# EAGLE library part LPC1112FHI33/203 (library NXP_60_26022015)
32-bit ARM Cortex-M0 microcontroller; up to 64 kB flash and 8 kB SRAM The LPC1110/11/12/13/14/15 are a ARM Cortex-M0 based, low-cost 32-bit MCU family, designed for 8/16-bit microcontroller applications, offering performance, low power, simple instruction set and memory addressing together with reduced code size compared to existing 8/16-bit architectures. The LPC1110/11/12/13/14/15 operate at CPU frequencies of up to 50 MHz. The peripheral complement of the LPC1110/11/12/13/14/15 includes up to 64 kB of flash memory, up to 8 kB of data memory, one Fast-mode Plus I 2 C-bus interface, one RS-485/EIA-485 UART, up to two SPI interfaces with SSP features, four general purpose counter/timers, a 10-bit ADC, and up to 42 general purpose I/O pins. Remark: The LPC111x series consists of the LPC1100 series (parts LPC111x/101/201/301), LPC1100L series (parts LPC111x/002/102/202/302), and the LPC1100XL series (parts LPC111x/103/203/303/323/333). The LPC1100L and LPC1100XL series include the power profiles, a windowed watchdog timer, and a configurable open-drain mode. AAL Eindhoven MK
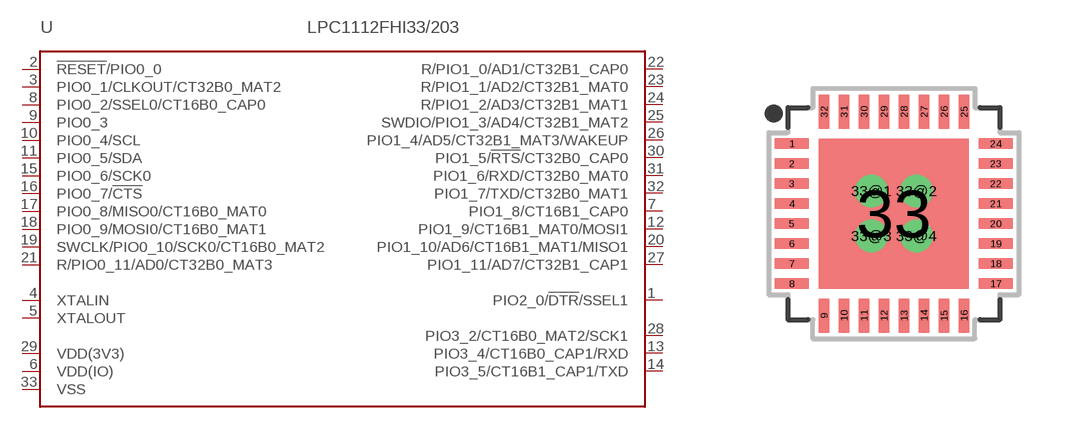
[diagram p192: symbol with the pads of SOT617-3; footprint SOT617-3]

Designator prefix U

## LPC1112FHI33/203 (ADC: 8; FLASH: 16kB; GPIO: 28; PWR_PROFILES: yes; SERIES: LPC1100XL; SPI: 2; SRAM: 4kB)  [SOT617-3]
1  PIO2_0/!DTR!/SSEL1
2  !RESET!/PIO0_0
3  PIO0_1/CLKOUT/CT32B0_MAT2
4  XTALIN  in
5  XTALOUT  out
6  VDD(IO)  pwr
7  PIO1_8/CT16B1_CAP0
8  PIO0_2/SSEL0/CT16B0_CAP0
9  PIO0_3
10  PIO0_4/SCL
11  PIO0_5/SDA
12  PIO1_9/CT16B1_MAT0/MOSI1
13  PIO3_4/CT16B0_CAP1/RXD
14  PIO3_5/CT16B1_CAP1/TXD
15  PIO0_6/SCK0
16  PIO0_7/!CTS!
17  PIO0_8/MISO0/CT16B0_MAT0
18  PIO0_9/MOSI0/CT16B0_MAT1
19  SWCLK/PIO0_10/SCK0/CT16B0_MAT2
20  PIO1_10/AD6/CT16B1_MAT1/MISO1
21  R/PIO0_11/AD0/CT32B0_MAT3
22  R/PIO1_0/AD1/CT32B1_CAP0
23  R/PIO1_1/AD2/CT32B1_MAT0
24  R/PIO1_2/AD3/CT32B1_MAT1
25  SWDIO/PIO1_3/AD4/CT32B1_MAT2
26  PIO1_4/AD5/CT32B1_MAT3/WAKEUP
27  PIO1_11/AD7/CT32B1_CAP1
28  PIO3_2/CT16B0_MAT2/SCK1
29  VDD(3V3)  pwr
30  PIO1_5/!RTS!/CT32B0_CAP0
31  PIO1_6/RXD/CT32B0_MAT0
32  PIO1_7/TXD/CT32B0_MAT1
33  VSS  pwr

## Footprint SOT617-3 (pad centres in mm)
SOT617-3 HVQFN32: plastic thermal enhanced very thin quad flat package; no leads; 32 terminals; body 5 x 5 x 0.85 mm JEDEC: MO-220 IEC: -- JEITA: --
smd 0.85 x 0.27: 1 -2.55,1.75; 2 -2.55,1.25; 3 -2.55,0.75; 4 -2.55,0.25; 5 -2.55,-0.25; 6 -2.55,-0.75; 7 -2.55,-1.25; 8 -2.55,-1.75; 17 2.55,-1.75; 18 2.55,-1.25; 19 2.55,-0.75; 20 2.55,-0.25; 21 2.55,0.25; 22 2.55,0.75; 23 2.55,1.25; 24 2.55,1.75
smd 0.27 x 0.85: 9 -1.75,-2.55; 10 -1.25,-2.55; 11 -0.75,-2.55; 12 -0.25,-2.55; 13 0.25,-2.55; 14 0.75,-2.55; 15 1.25,-2.55; 16 1.75,-2.55; 25 1.75,2.55; 26 1.25,2.55; 27 0.75,2.55; 28 0.25,2.55; 29 -0.25,2.55; 30 -0.75,2.55; 31 -1.25,2.55; 32 -1.75,2.55
smd 3.75 x 3.75: 33 0,0
drill 0.3 pad 0.6: 33@1 -0.562,0.562; 33@2 0.562,0.562; 33@3 -0.562,-0.562; 33@4 0.562,-0.562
